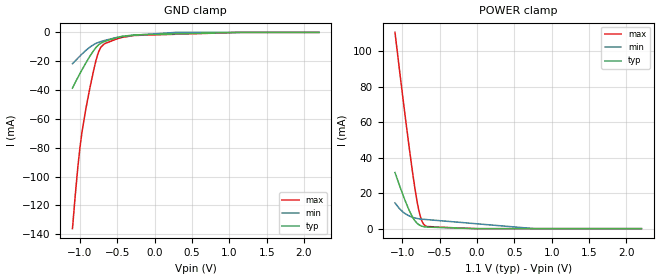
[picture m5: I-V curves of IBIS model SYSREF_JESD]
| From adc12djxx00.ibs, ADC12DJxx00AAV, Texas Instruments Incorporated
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|   Model SYSREF_JESD
[Model]   SYSREF_JESD
Model_type   Input
Vinl = .57
Vinh = 1.33
|   typ   min   max
|   (nom PVT)   (slow PVT)   (fast PVT)
C_comp   0.996p   0.974p   1.029p
[Voltage Range]   1.1   1.05   1.15
[Temperature Range]   27   125   -40
[Power Clamp Reference]   1.1   1.05   1.15
[GND Clamp Reference]   0   0   0
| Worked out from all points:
|   POWER clamp passes 1 mA (typ) near -0.70 V on its own axis
[GND Clamp]
|   Voltage   I(typ)   I(min)   I(max)
-1.1V     -38.65mA   -21.76mA   -136.1mA
-1.031V   -31.52mA   -18mA      -94.8mA
-1.001V   -28.65mA   -16.45mA   -80.38mA
-968mV    -25.53mA   -14.77mA   -67.54mA
-928.4mV  -21.89mA   -12.86mA   -55.25mA
-862.4mV  -16.15mA   -10.03mA   -37.42mA
-783.2mV  -10.36mA   -7.587mA   -19.11mA
-720.5mV  -7.508mA   -6.363mA   -10.3mA
-677.6mV  -6.432mA   -5.693mA   -8.125mA
-275mV    -1.751mA   -1.996mA   -2.151mA
279.4mV   -1.031mA   -523.7nA   -1.295mA
2.2V      0A         0A         0A
[POWER Clamp]
|   Voltage   I(typ)   I(min)   I(max)
-1.1V     31.7mA     14.51mA    110.8mA
-1.041V   24.54mA    11.35mA    89.92mA
-964.7mV  15.91mA    8.507mA    63.93mA
-911.9mV  10.53mA    7.24mA     46.55mA
-836mV    4.622mA    6.061mA    23.62mA
-793.1mV  2.662mA    5.673mA    12.89mA
-753.5mV  1.62mA     5.439mA    5.872mA
-717.2mV  1.137mA    5.278mA    2.54mA
-694.1mV  983.7uA    5.188mA    1.628mA
-1.1mV    2.316uA    2.743mA    4.374uA
767.8mV   0A         9.468uA    0A
2.2V      0A         0A         0A
